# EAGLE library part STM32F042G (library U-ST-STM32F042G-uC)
STM32 Microcontroller http://www.st.com/content/st_com/en/products/microcontrollers/stm32-32-bit-arm-cortex-mcus.html?querycriteria=productId=SC1169
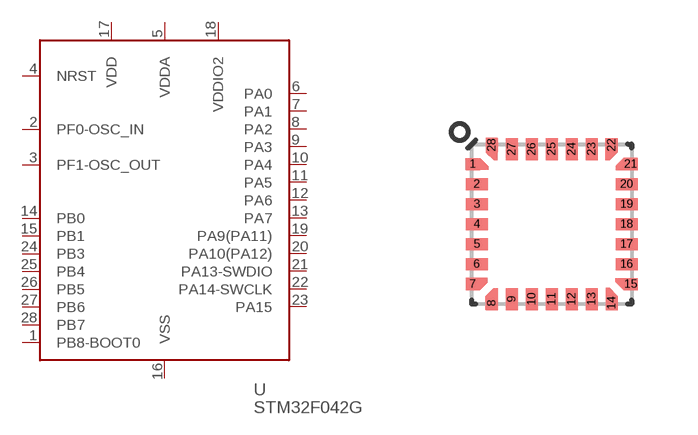
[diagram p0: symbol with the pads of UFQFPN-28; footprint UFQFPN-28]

Designator prefix -

## STM32F042G  [UFQFPN-28]
1  PB8-BOOT0
2  PF0-OSC_IN
3  PF1-OSC_OUT
4  NRST
5  VDDA  pwr
6  PA0
7  PA1
8  PA2
9  PA3
10  PA4
11  PA5
12  PA6
13  PA7
14  PB0
15  PB1
16  VSS  pwr
17  VDD  pwr
18  VDDIO2  pwr
19  PA9(PA11)
20  PA10(PA12)
21  PA13-SWDIO
22  PA14-SWCLK
23  PA15
24  PB3
25  PB4
26  PB5
27  PB6
28  PB7

## Footprint UFQFPN-28 (pad centres in mm)
QFPN-28 7x7 x 1.8mm Source: http://www.st.com/stonline/products/literature/ds/11115/lis3lv02dq.pdf
smd 0.35 x 0.3: 1 -1.975,1.5; 7 -1.975,-1.5; 15 1.975,-1.5; 21 1.975,1.5
smd 0.55 x 0.3: 2 -1.875,1; 3 -1.875,0.5; 4 -1.875,0; 5 -1.875,-0.5; 6 -1.875,-1; 16 1.875,-1; 17 1.875,-0.5; 18 1.875,0; 19 1.875,0.5; 20 1.875,1
smd 0.3 x 0.35: 8 -1.5,-1.975; 14 1.5,-1.975; 22 1.5,1.975; 28 -1.5,1.975
smd 0.3 x 0.55: 9 -1,-1.875; 10 -0.5,-1.875; 11 0,-1.875; 12 0.5,-1.875; 13 1,-1.875; 23 1,1.875; 24 0.5,1.875; 25 0,1.875; 26 -0.5,1.875; 27 -1,1.875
